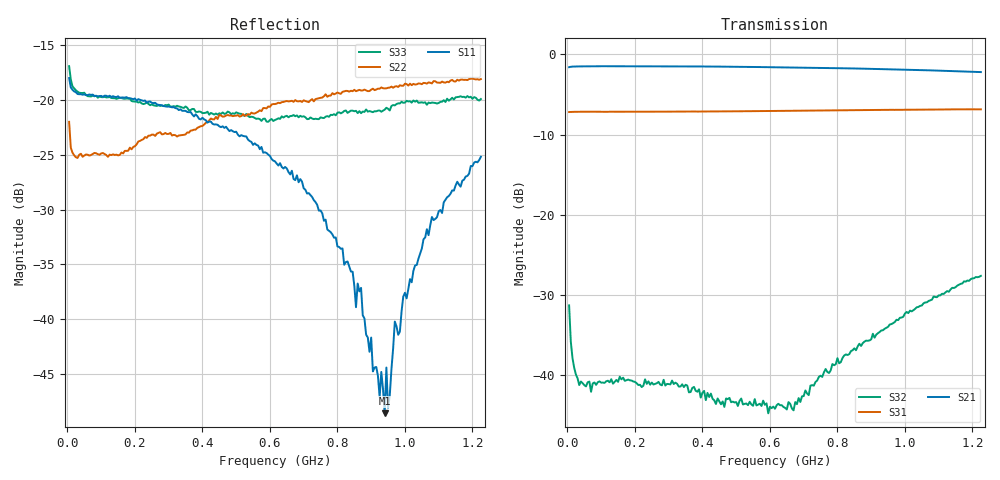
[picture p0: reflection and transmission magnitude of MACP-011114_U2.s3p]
!Agilent Technologies,E5071C,MY46110647,A.11.31
!Date: Tue Jan 09 14:59:50 2024 DD
!Data & Calibration Information:
!MACP-011114 soldered onto PT-0030145 with F connectors, calibration PCB PT-0003653. Port1 (pin1) Port2 (pin6) Port3 (pin3)
!Freq	S11:SOLT3(ON)	S12:SOLT3(ON)	S13:SOLT3(ON)
!	S21:SOLT3(ON)	S22:SOLT3(ON)	S23:SOLT3(ON)
!	S31:SOLT3(ON)	S32:SOLT3(ON)	S33:SOLT3(ON)
!PortZ  Port1:75+j0  Port2:75+j0  Port3:75+j0
!Above PortZ is port z conversion or system Z0 setting when saving the data.
!When reading, reference impedance value at option line is always used.
# Hz S MA R 75
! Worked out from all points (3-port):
!   245 points, 5 MHz to 1.225 GHz, reference 75 ohm
!   strongest paths, dB at 5 MHz, 310 MHz, 615 MHz, 920 MHz, 1.225 GHz:
!     S21: -1.6, -1.5, -1.6, -1.8, -2.2
!     S31: -7.2, -7.1, -7.1, -6.9, -6.8
!     S32: -31.3, -40.7, -44.2, -34.8, -27.6
!   lowest |S11| = -48.6 dB at 940 MHz (marker M1), VSWR 1.01, Z = 74.7 - j0.445 ohm
!   |S11| at or under -10 dB: start of sweep to end of sweep
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5000000  0.126 160.0  0.8348 2.8  0.4371 -178.7
         0.8331 2.8  0.07953 64.1  0.02501 96.9
         0.4373 -178.9  0.02719 92.6  0.1427 151.9
2.5e7  0.1085 173.9  0.8419 -0.4  0.4387 178.2
       0.8415 -0.3  0.05483 15.3  0.009945 46.0
       0.4389 178.1  0.01009 50.5  0.1107 168.2
7e7  0.1055 174.4  0.8441 -2.9  0.4393 173.7
     0.8441 -2.9  0.0561 -0.8  0.009772 23.7
     0.4391 173.7  0.007858 26.3  0.1038 168.9
6.15e8  0.05249 144.2  0.8315 -29.5  0.4443 123.6
        0.8325 -29.3  0.09582 -48.8  0.004247 55.1
        0.4437 123.6  0.006159 59.1  0.08111 112.0
8.7e8  0.01389 147.4  0.8145 -42.2  0.4496 100.0
       0.8162 -42.0  0.1105 -55.6  0.01557 97.4
       0.4493 99.9  0.01518 91.7  0.08708 81.6
9.4e8  0.003718 -126.7  0.8086 -45.7  0.4512 93.5
       0.8102 -45.7  0.1129 -59.3  0.01928 95.7
       0.4513 93.3  0.01943 89.9  0.09036 69.8
9.45e8  0.006014 -112.7  0.8081 -46.0  0.4513 93.0
        0.8097 -45.9  0.1131 -59.6  0.01928 95.4
        0.4509 92.9  0.0197 90.3  0.09218 68.7
9.7e8  0.009752 -100.0  0.806 -47.3  0.4514 90.6
       0.8072 -47.2  0.1152 -61.0  0.02066 93.7
       0.4513 90.5  0.02141 88.1  0.09451 66.8
1.065e9  0.02572 -97.1  0.7961 -52.3  0.4534 81.5
         0.7972 -52.2  0.1188 -65.4  0.02805 89.1
         0.4532 81.4  0.02841 84.4  0.09514 58.6
1.225e9  0.05507 -106.9  0.7751 -61.0  0.4556 65.9
         0.7764 -60.8  0.1246 -78.4  0.04003 75.9
         0.4547 65.7  0.04155 73.0  0.1011 44.1
